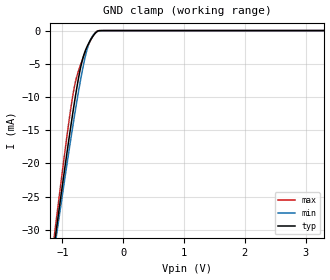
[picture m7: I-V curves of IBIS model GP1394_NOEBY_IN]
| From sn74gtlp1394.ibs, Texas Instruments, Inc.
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[Model]   GP1394_NOEBY_IN
Model_type  Input
Vinl=0.8
Vinh=2.0
| variable   typ   min   max
C_comp   2.79pF   1.98pF   3.98pF
[Temperature Range]   40   100   -40
| Ambient temperature   25   85   -40
[Voltage range]   3.3   3.15   3.45
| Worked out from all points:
|   GND clamp passes 1 mA (typ) near -0.51 V on its own axis
[GND Clamp]
| GP1394_NOEBY_IN
|   Voltage   I(typ)   I(min)   I(max)
-5.5V     -355mA     -335.7mA   -380.8mA
-1.155V   -33.69mA   -34.48mA   -32.48mA
-1.115V   -30.96mA   -31.93mA   -29.51mA
-1.075V   -28.26mA   -29.39mA   -26.57mA
-895mV    -16.45mA   -18.27mA   -13.82mA
-840mV    -13.04mA   -15.02mA   -10.38mA
-795mV    -10.38mA   -12.44mA   -8.1mA
-690mV    -5.112mA   -6.847mA   -4.848mA
-605mV    -2.629mA   -3.201mA   -2.83mA
-535mV    -1.376mA   -1.322mA   -1.427mA
-445mV    -270.8uA   -216.6uA   -189uA
3.3V      184.4pA    833.1pA    1.235nA
